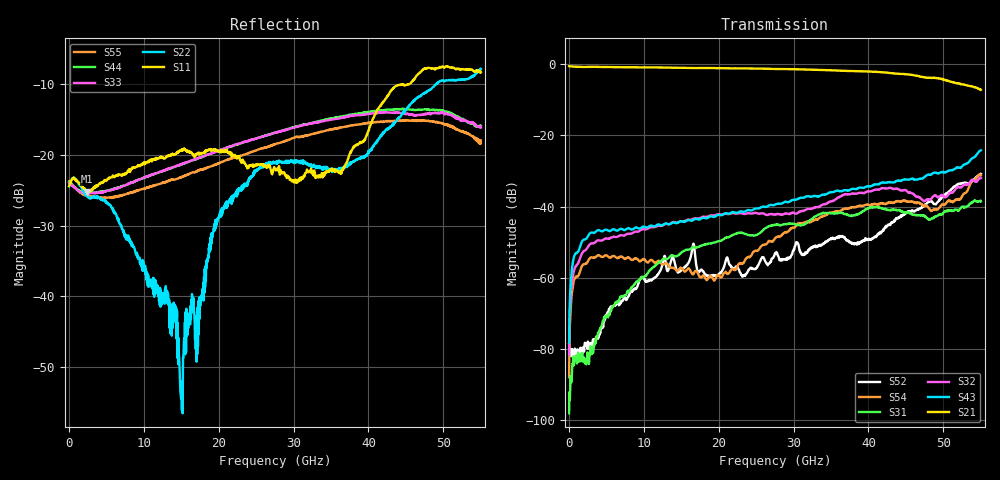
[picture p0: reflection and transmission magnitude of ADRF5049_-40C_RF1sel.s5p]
! Device  : ADRF5049
! Description: Silicon SP4T Switch Non-Reflective
! Frequency:  9kHz -  45 GHz
! Ports:
!  RFC = Port 1
!  RF1 = Port 2
!  RF2 = Port 3
!	 RF3 = Port 4
!  RF4 = Port 5
! VSS  =  +3.30 Volts
! VDD  =  -3.30 Volts
! EN  =  0.00 Volts
! LS  =  0.00 Volts
! V1  =  0.00 Volts
! V2  =  0.00 Volts
! Data:  Data was collected using an calibrated 4 port network analyzer.
! Notes: Analog Devices supplies this data as a sample of measured data
!  for this product.  Your particular data for this product may vary.
!  Data was taken at -40C degrees C.
!  Analog Devices reserves the right to change this data at anytime.
# hz S db R 50
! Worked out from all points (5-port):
!   1100 points, 50 MHz to 55 GHz, reference 50 ohm
!   strongest paths, dB at 50 MHz, 13.8 GHz, 27.55 GHz, 41.3 GHz, 55 GHz:
!     S21: -0.6, -1.0, -1.4, -2.2, -7.2
!     S43: -78.2, -44.6, -39.5, -33.8, -24.2
!     S32: -81.5, -44.5, -42.2, -35.2, -32.0
!     S31: -98.1, -53.7, -45.1, -40.3, -38.5
!     S54: -87.9, -57.2, -48.8, -39.2, -31.2
!     S52: -78.7, -54.5, -53.1, -47.6, -30.8
!   lowest |S11| = -25.2 dB at 2.45 GHz (marker M1), VSWR 1.12, Z = 54.8 - j3.17 ohm
!   |S11| at or under -10 dB: start of sweep to 44.39 GHz; 44.40974 GHz to 44.4856 GHz (75.86 MHz wide, 0.171 % of centre); 44.6 GHz to 45.2 GHz (600.3 MHz wide, 1.34 % of centre)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
